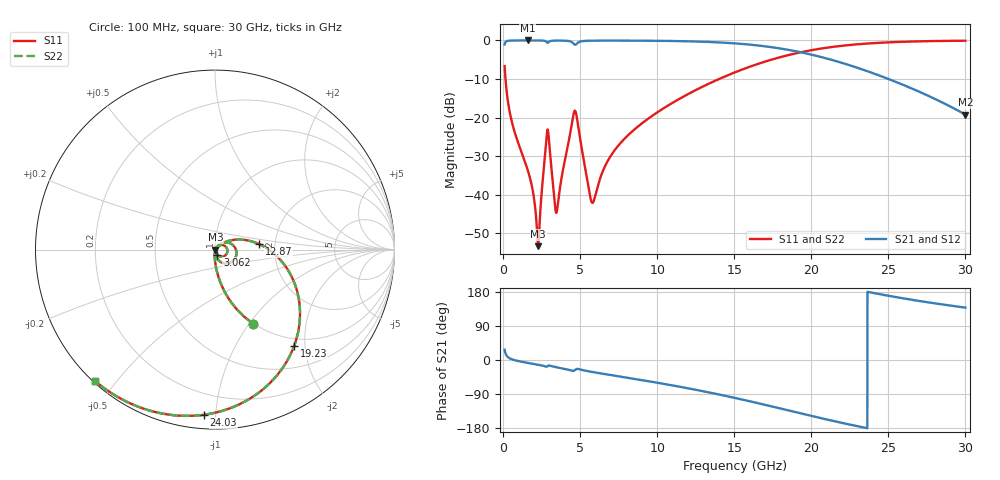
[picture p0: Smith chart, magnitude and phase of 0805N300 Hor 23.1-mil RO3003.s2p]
# GHz S MA R 50
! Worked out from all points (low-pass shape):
!   3201 points, 100 MHz to 30 GHz, reference 50 ohm
!   highest |S21| = -0.01 dB at 1.614 GHz (marker M1); lowest = -19.2 dB at 30 GHz (marker M2)
!   |S21| within 3 dB of the highest: start of sweep to 19.24 GHz
!   lowest |S11| = -53.3 dB at 2.277 GHz (marker M3), VSWR 1.00, Z = 50.2 - j0.0769 ohm
!   |S11| at or under -10 dB: 157.1 MHz to 14.02 GHz (13.86 GHz wide, 196 % of centre)
!   |S22| runs from -53.3 to -0.1 dB; largest |S21 - S12| = 0
!   S11 on the Smith chart (normalised r, x): 100 MHz: 0.99, -1.04; 3.062 GHz: 1.03, -0.06; 12.87 GHz: 1.65, +0.11; 19.23 GHz: 0.85, -1.78; 24.03 GHz: 0.08, -0.93; 30 GHz: 0.01, -0.44
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0.1  0.4645 -62.8  0.8852 27.1  0.8852 27.1  0.4645 -62.8
0.5765313  0.08708 -87.8  0.9955 1.8  0.9955 1.8  0.08708 -87.8
1.613687  0.02047 -94.5  0.9986 -7.7  0.9986 -7.7  0.02047 -94.5
2.277094  0.002158 -20.8  0.9978 -12.5  0.9978 -12.5  0.002158 -20.8
2.809687  0.05376 26.3  0.9605 -17.6  0.9605 -17.6  0.05376 26.3
2.931156  0.06445 -32.9  0.9384 -15.0  0.9384 -15.0  0.06445 -32.9
3.061969  0.03239 -65.7  0.9789 -15.4  0.9789 -15.4  0.03239 -65.7
3.323594  0.008849 -55.8  0.9929 -17.9  0.9929 -17.9  0.008849 -55.8
3.46375  0.005856 -6.6  0.9942 -19.1  0.9942 -19.1  0.005856 -6.6
4.594344  0.1154 1.9  0.8985 -28.5  0.8985 -28.5  0.1154 1.9
4.771875  0.1044 -47.3  0.9033 -23.7  0.9033 -23.7  0.1044 -47.3
5.089563  0.04129 -79.3  0.9746 -25.9  0.9746 -25.9  0.04129 -79.3
5.827719  0.00791 -13.5  0.9923 -31.9  0.9923 -31.9  0.00791 -13.5
7.219938  0.03728 41.5  0.9943 -41.2  0.9943 -41.2  0.03728 41.5
10.06978  0.1192 27.3  0.9877 -60.4  0.9877 -60.4  0.1192 27.3
12.87291  0.2473 7.1  0.9626 -81.5  0.9626 -81.5  0.2473 7.1
15.05  0.386 -11.1  0.9149 -100.1  0.9149 -100.1  0.386 -11.1
19.22666  0.6959 -50.8  0.7081 -140.0  0.7081 -140.0  0.6959 -50.8
20.03956  0.749 -58.6  0.652 -147.9  0.652 -147.9  0.749 -58.6
24.02934  0.922 -93.8  0.3745 176.9  0.3745 176.9  0.922 -93.8
25.01978  0.9442 -101.3  0.3157 169.4  0.3157 169.4  0.9442 -101.3
30  0.9914 -132.6  0.1092 138.3  0.1092 138.3  0.9914 -132.6
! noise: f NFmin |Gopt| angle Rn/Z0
0.1  0.0004743  0.8724  0.8331  0.0008016
3.417  0.01079  0.8154  18.77  0.01189
6.743  0.01395  0.7359  36.47  0.009542
10.06  0.01648  0.6853  53.01  0.008208
13.39  0.02152  0.6888  68.47  0.009331
16.7  0.02855  0.7135  82.87  0.01129
20.03  0.03901  0.7531  96.58  0.01447
23.35  0.05594  0.8039  109.9  0.02001
26.67  0.08745  0.8616  123.2  0.03121
30  0.1601  0.9194  136.7  0.06052
